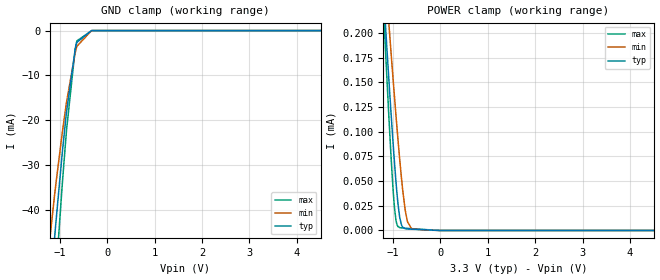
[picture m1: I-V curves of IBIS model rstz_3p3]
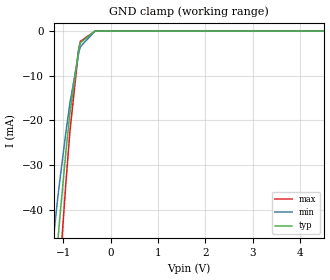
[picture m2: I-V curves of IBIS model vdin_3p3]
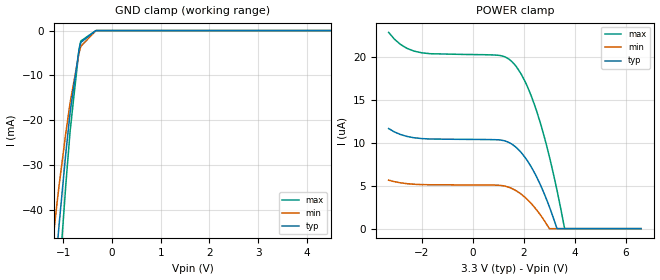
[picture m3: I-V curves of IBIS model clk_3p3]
|Texas Instruments Incorporated
| QVGA Sensor with Digital Output
| Marketing part#   Digital Voltage Range   Package-type   #pins
| OPT8241BGA   1.7V-3.6V   BGA   78
[IBIS Ver]   4.1
[File name]   opt8241.ibs
[File Rev]   2.0
[Date]   1/08/2016
[Source]
| Texas Instruments Incorporated.
| Analog-eLab Design Center, HPA
| 12500 TI Blvd
| Dallas, TX -75243
[Notes]   Revision History:
| Rev 3.0: 1/08/2016
| - clkout_fast_*,clkout_slow_*,clkout_hiz_* models generated at 50MHz.
| - illum_fast,illum_fastest,illum_slowest models generated at 80MHz.
| Rev 2.0: 5/28/2015
| - lvds model regenerated at 300MHz.
| Rev 1.0: 5/14/2015
| - Initial version of the model
| - Model generated from simulations in TISPICE
| - Model matched to SPICE simulation
| - C_comp although listed in numerical order of value are
|   obtained from varying PVT conditions. For PVT conditions for
|   each specific value refer the buffer description under
|   respective [Model]. IBIS model user is responsible for using
|   appropriate C_comp to simulate for Signal Integrity.
|* EXCEPTION:   *
|* - For models clk_*,There will be a leakage current in the POWER   *
|*   clamp I-V Table because of two resistors(R0 & R1) connected to Pad.*
|* - For model illum,There will be a leakage current in the POWER clamp *
|*   I-V Table because of two resistors(R0 & R1) connected to Pad.   *
|* - For models rstz_*,There will be a leakage current in GND clamp I-V *
|*   Table because of two resistors network(R0 & R1) connected to Pad.  *
|* - For lvds, Pullup and Pulldown will not pass through zero due to   *
|*   driver switch(MPSWP_TX and MNSWP_TX) arrangement.   *
[Disclaimer]
| This model is designed as an aid for customers of Texas Instruments.
| TI and its licensors and suppliers make no warranties, either expressed
| or implied, with respect to this  model, including the warranties of
| merchantability or fitness for a particular purpose. The model is
| provided solely on an "as is" basis. The entire risk as to its quality
| and performance is with the customer.
[Copyright]
(C) Copyright 2015 Texas Instruments Incorporated.All rights reserved.
|   OPT8241BGA
[Component]   OPT8241BGA
[Manufacturer]   TI
[Package]   |78 BGA package
|   typ   min   max
R_pkg   0.0712   0.0262   0.1046
L_pkg   0.9785nH   0.5979nH   1.4931nH
C_pkg   0.3322pF   0.3071pF   0.4589pF
[Pin]  signal_name   model_name   R_pin   L_pin   C_pin
A1   NC   nc   na   na   na
A2   GPO<0>   gpo   na   na   na
A3   SDATA   sclkdata   na   na   na
A4   GND   gnd   na   na   na
A5   VMIXH   power   na   na   na
A6   VMIXH   power   na   na   na
A7   GND   gnd   na   na   na
A8   GND   gnd   na   na   na
A9   VMIXH   power   na   na   na
A10   VMIXH   power   na   na   na
A11   GND   gnd   na   na   na
A12   ILLUM_P   illum_pn   na   na   na
A13   ILLUM_N   illum_pn   na   na   na
A14   DVDDH   power   na   na   na
A15   GND   gnd   na   na   na
A16   ILLUM_EN   illumen   na   na   na
A17   AVDDH   power   na   na   na
A18   AVDD_PLL   power   na   na   na
A19   NC   nc   na   na   na
B1   GPO<1>   gpo   na   na   na
B3   SCLK   sclkdata   na   na   na
B17   FSC   power   na   na   na
B19   MCLK   clk   na   na   na
C1   VD_IN   vdin   na   na   na
C3   RSTZ   rstz   na   na   na
C17   NC   nc   na   na   na
C19   DMOD_CLK   clk   na   na   na
D1   HD_QD   vd   na   na   na
D3   AVDD   power   na   na   na
D17   RFU   nc   na   na   na
D19   TP2   nc   na   na   na
E1   VD_QD   vd   na   na   na
E3   AVSS   gnd   na   na   na
E17   PVDD   power   na   na   na
E19   QPORT   nc   na   na   na
F1   VD_FR   vd   na   na   na
F3   REFM   nc   na   na   na
F17   AVSS_PLL   gnd   na   na   na
F19   DVDD   power   na   na   na
G1   IOVSS   gnd   na   na   na
G3   REFP   nc   na   na   na
G17   AVDD   power   na   na   na
G19   DVSS   gnd   na   na   na
H1   IOVDD   power   na   na   na
H3   AVSS   gnd   na   na   na
H17   AVSS   gnd   na   na   na
H19   DVDD   power   na   na   na
J1   CMOS<14>   clkout   na   na   na
J3   VD_SF   vd   na   na   na
J17   TP1   nc   na   na   na
J19   SUM_M   lvds   na   na   na
K1   CMOS<13>   clkout   na   na   na
K3   CMOS<15>   clkout   na   na   na
K17   SUM_P   lvds   na   na   na
K19   DIFF1_M   lvds   na   na   na
L1   CMOS<12>   clkout   na   na   na
L3   CMOS<11>   clkout   na   na   na
L17   DIFF1_P   lvds   na   na   na
L19   DCLKM   lvds   na   na   na
M1   NC   nc   na   na   na
M2   CMOS<10>   clkout   na   na   na
M3   CMOS<9>   clkout   na   na   na
M4   CMOS<8>   clkout   na   na   na
M5   CLKOUT   clkout   na   na   na
M6   CMOS<7>   clkout   na   na   na
M7   CMOS<6>   clkout   na   na   na
M8   CMOS<5>   clkout   na   na   na
M9   CMOS<4>   clkout   na   na   na
M10   CMOS<3>   clkout   na   na   na
M11   CMOS<2>   clkout   na   na   na
M12   CMOS<1>   clkout   na   na   na
M13   CMOS<0>   clkout   na   na   na
M14   PCLK_P   lvds   na   na   na
M15   PCLK_M   lvds   na   na   na
M16   DIFF0_P   lvds   na   na   na
M17   DIFF0_M   lvds   na   na   na
M18   DCLKP   lvds   na   na   na
M19   NC   nc   na   na   na
[Diff_pin]   inv_pin   vdiff   tdelay_typ   tdelay_min   tdelay_max
K17   J19   NA   0   0   0
L17   K19   NA   0   0   0
M14   M15   NA   0   0   0
M16   M17   NA   0   0   0
M18   L19   NA   0   0   0
|   Model Selectors
[Model Selector] rstz
rstz_1p8   1.8V   digital Input
rstz_3p3   3.3V   digital Input
[Model Selector] vdin
vdin_1p8   1.8V   digital Input
vdin_3p3   3.3V   digital Input
[Model Selector] clk
clk_1p8   1.8V   digital Input
clk_3p3   3.3V   digital Input
[Model Selector] gpo
gpo_1p8   1.8V   digital Output
gpo_3p3   3.3V   digital Output
[Model Selector] clkout
clkout_1p8   1.8V   digital Output
clkout_3p3   3.3V   digital Output
clkout_fast_1p8  1.8V   digital Output
clkout_fast_3p3  1.8V   digital Output
clkout_slow_1p8  1.8V   digital Output
clkout_slow_3p3  1.8V   digital Output
clkout_hiz_1p8   1.8V   digital 3-state
clkout_hiz_3p3   1.8V   digital 3-state
[Model Selector] illum_pn
illum   3.3V   digital IO
illum_fast   3.3V   digital IO
illum_fastest   3.3V   digital IO
illum_slowest   3.3V   digital IO
[Model Selector] vd
vd_1p8   1.8V   digital IO
vd_3p3   3.3V   digital IO
[Model Selector] sclkdata
sclkdata_1p8   1.8V   digital IO_open_drain
sclkdata_3p3   3.3V   digital IO_open_drain
| Models and submodels in the file (26): rstz_1p8 (Input), rstz_3p3 (Input), vdin_1p8 (Input), vdin_3p3 (Input), clk_1p8 (Input), clk_3p3 (Input), gpo_1p8 (Output), gpo_3p3 (Output), illumen (Output), clkout_1p8 (Output), clkout_3p3 (Output), clkout_fast_1p8 (Output), clkout_fast_3p3 (Output), clkout_slow_1p8 (Output), clkout_slow_3p3 (Output), clkout_hiz_1p8 (3-state), clkout_hiz_3p3 (3-state), vd_1p8 (I/O), vd_3p3 (I/O), illum (I/O), illum_fast (I/O), illum_fastest (I/O), illum_slowest (I/O), sclkdata_1p8 (I/O_open_drain), sclkdata_3p3 (I/O_open_drain), lvds (Output)
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|   rstz_3p3 Model
[Model]   rstz_3p3
Model_type   Input
Vinl = 0.99
Vinh = 2.31
|   typ   min   max
|   (nom PVT)   (fast PVT)   (slow PVT)
C_comp   2.023e-12   1.832e-12   2.219e-12
[Model spec]
|subparameter
Vinl   0.99   0.90   1.08
Vinh   2.31   2.10   2.52
| Where nom  PVT is Nominal Process, 3.3V, 27C
|   Fast PVT is Strong Process,  3.6V, -40C
|   Slow PVT is Weak Process,   3V, 125C
[Voltage Range]   3.3   3   3.6
|Junction Temperature
[Temperature Range]   27   125   -40
[Power Clamp Reference]   3.3   3   3.6
[GND Clamp Reference]   0   0   0
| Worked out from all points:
|   POWER clamp passes 1 mA (typ) near -2.11 V on its own axis
[GND Clamp]
|   Voltage   I(typ)   I(min)   I(max)
-3.3V     -1.622A    -1.413A    -1.789A
-1.467V   -94.33mA   -71.79mA   -120.1mA
-1.111V   -46.47mA   -36.85mA   -59.33mA
-1.079V   -42.52mA   -33.96mA   -54.21mA
-947.1mV  -27.27mA   -22.78mA   -34.28mA
-858mV    -18.14mA   -15.99mA   -22.25mA
-675mV    -4.21mA    -4.973mA   -4.156mA
-639.6mV  -2.625mA   -3.51mA    -2.314mA
-330mV    -3.16uA    -13.25uA   -3.645uA
6.6V      0A         0A         0A
[POWER Clamp]
|   Voltage   I(typ)   I(min)   I(max)
-3.3V     2.003mA    1.737mA    2.501mA
-1.206V   246.5uA    288.6uA    232.4uA
-1.164V   213.5uA    260.9uA    190.7uA
-1.133V   189.3uA    240.5uA    160.4uA
-1.082V   151uA      208uA      113.1uA
-966.9mV  69.18uA    135.7uA    23.51uA
-920.7mV  41.3uA     108.2uA    7.22uA
-854.7mV  12.85uA    71.23uA    2.892uA
-739.2mV  1.82uA     20.26uA    2.305uA
-693.6mV  1.541uA    9.038uA    2.151uA
-606mV    1.302uA    1.737uA    1.861uA
6.6V      0A         0A         0A
|   vdin_3p3 Model
[Model]   vdin_3p3
Model_type   Input
Vinl = 0.99
Vinh = 2.31
|   typ   min   max
|   (nom PVT)   (fast PVT)   (slow PVT)
C_comp   2.023e-12   1.832e-12   2.219e-12
[Model spec]
|subparameter
Vinl   0.99   0.90   1.08
Vinh   2.31   2.10   2.52
| Where nom  PVT is Nominal Process, 3.3V, 27C
|   Fast PVT is Strong Process,  3.6V, -40C
|   Slow PVT is Weak Process,   3V, 125C
[Voltage Range]   3.3   3   3.6
|Junction Temperature
[Temperature Range]   27   125   -40
[Power Clamp Reference]   3.3   3   3.6
[GND Clamp Reference]   0   0   0
[GND Clamp]
|   Voltage   I(typ)   I(min)   I(max)
-3.3V     -1.673A    -1.458A    -1.843A
-1.47V    -94.75mA   -72.1mA    -120.6mA
-1.115V   -46.92mA   -37.17mA   -59.9mA
-1.082V   -42.92mA   -34.25mA   -54.73mA
-947.1mV  -27.27mA   -22.78mA   -34.28mA
-858mV    -18.14mA   -15.99mA   -22.25mA
-678mV    -4.363mA   -5.108mA   -4.34mA
-639.6mV  -2.623mA   -3.509mA   -2.311mA
-330mV    -981.6nA   -11.94uA   -87.51nA
6.6V      0A         0A         0A
[POWER Clamp]
|   Voltage   I(typ)   I(min)   I(max)
-3.3V     0A         0A         0A
0V        0A         0A         0A
6.6V      0A         0A         0A
|   clk_3p3 Model
[Model]   clk_3p3
Model_type   Input
Vinl = 0.99
Vinh = 2.31
|   typ   min   max
|   (nom PVT)   (fast PVT)   (slow PVT)
C_comp   2.023e-12   1.842e-12   2.219e-12
[Model spec]
|subparameter
Vinl   0.99   0.90   1.08
Vinh   2.31   2.10   2.52
| Where nom  PVT is Nominal Process, 3.3V, 27C
|   Fast PVT is Strong Process,  3.6V, -40C
|   Slow PVT is Weak Process,   3V, 125C
[Voltage Range]   3.3   3   3.6
|Junction Temperature
[Temperature Range]   27   125   -40
[Power Clamp Reference]   3.3   3   3.6
[GND Clamp Reference]   0   0   0
[GND Clamp]
|   Voltage   I(typ)   I(min)   I(max)
-3.3V     -1.673A    -1.458A    -1.843A
-1.47V    -94.76mA   -72.1mA    -120.6mA
-1.115V   -46.93mA   -37.17mA   -59.91mA
-1.082V   -42.93mA   -34.26mA   -54.74mA
-947.1mV  -27.27mA   -22.78mA   -34.29mA
-858mV    -18.15mA   -15.99mA   -22.25mA
-678mV    -4.368mA   -5.111mA   -4.349mA
-639.6mV  -2.628mA   -3.512mA   -2.32mA
-330mV    -4.192uA   -13.68uA   -5.628uA
6.6V      0A         0A         0A
[POWER Clamp]
|   Voltage   I(typ)   I(min)   I(max)
-3.3V     11.68uA    5.659uA    22.9uA
-2.836V   10.99uA    5.349uA    21.5uA
-2.289V   10.6uA     5.18uA     20.71uA
1.02V     10.36uA    5.062uA    20.23uA
1.452V    10uA       4.786uA    19.7uA
1.931V    8.763uA    3.946uA    17.85uA
2.241V    7.451uA    3.092uA    15.87uA
2.507V    6.008uA    2.168uA    13.68uA
3.003V    2.546uA    0A         8.395uA
3.303V    0A         0A         4.447uA
3.598V    0A         0A         38.14nA
6.6V      0A         0A         0A
